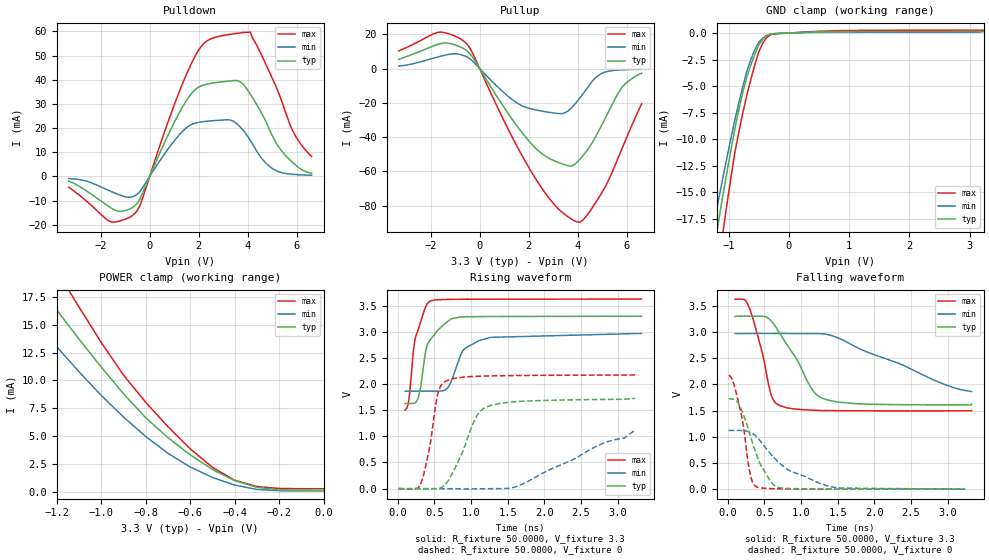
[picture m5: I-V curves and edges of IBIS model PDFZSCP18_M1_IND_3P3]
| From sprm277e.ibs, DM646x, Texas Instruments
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|   Model Cell PDFZSCP18_M1_IND_3P3
[Model]   PDFZSCP18_M1_IND_3P3
Model_type   I/O
Polarity   Non-Inverting
Enable   Active-Low
Vinl =  0.8V
Vinh =  2V
Cref =  10.0000pF
Rref =  50.0000
Vref =  1.5V
Vmeas =  1.65
C_comp   1.471252p   1.436302p   1.510805p
[Model Spec]
Vinl   0.8V   0.8V   0.8V
Vinh   2V   2V   2V
[Temperature Range]   25   125   -40
[Voltage Range]   3.3   2.97   3.63
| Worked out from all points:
|   slope of the pulldown table from 0 to 0.495 V, typ, clamps not added: 42.9 ohm
|   slope of the pullup table from 0 to 0.495 V, typ, clamps not added: 42.8 ohm
|   GND clamp passes 1 mA (typ) near -0.48 V on its own axis
|   POWER clamp passes 1 mA (typ) near -0.40 V on its own axis
|   rising waveform, R_fixture 50.0000, V_fixture 3.3: 20-80 % time 194ps typ, 261ps min, 145ps max; typ from 1.63 V to 3.3 V
|   rising waveform, R_fixture 50.0000, V_fixture 0: 20-80 % time 311ps typ, 973ps min, 153ps max; typ from 0 V to 1.73 V
|   falling waveform, R_fixture 50.0000, V_fixture 3.3: 20-80 % time 410ps typ, 1.11ns min, 214ps max; typ from 3.3 V to 1.63 V
|   falling waveform, R_fixture 50.0000, V_fixture 0: 20-80 % time 274ps typ, 623ps min, 153ps max; typ from 1.73 V to 0 V
[POWER_clamp]
|   voltage   I(typ)   I(min)   I(max)
-3.3V     84.79mA    64.06mA    102.5mA
-1.4V     21.98mA    17.8mA     26.67mA
-1.367V   21.02mA    17mA       25.54mA
-1.233V   17.27mA    13.84mA    21.04mA
-1.133V   14.62mA    11.55mA    17.73mA
-900mV    8.821mA    6.72mA     10.51mA
-800mV    6.658mA    4.97mA     8.044mA
-600mV    3.315mA    2.217mA    3.857mA
-500mV    1.994mA    1.273mA    2.187mA
-400mV    987.1uA    584.8uA    1.02mA
-300mV    389.1uA    194.4uA    453.4uA
0V        136.1uA    62.81uA    257uA
[Pulldown]
|   voltage   I(typ)   I(min)   I(max)
-3.3V     -1.945mA   -836.9uA   -4.474mA
-1.6V     -12.83mA   -6.075mA   -18.69mA
-600mV    -12.09mA   -8.013mA   -15.3mA
1.1V      24.29mA    15.95mA    32.25mA
1.9V      36.3mA     22.19mA    50.64mA
2.5V      38.52mA    23.01mA    56.95mA
3.3V      39.52mA    23.34mA    58.83mA
3.8V      38.23mA    19.26mA    59.54mA
4.1V      34.11mA    14.97mA    59.73mA
5V        16.81mA    3.301mA    40.55mA
5.9V      5.118mA    845.8uA    17.51mA
6.6V      1.393mA    503uA      8.266mA
[Pullup]
|   voltage   I(typ)   I(min)   I(max)
-3.3V     5.393mA    1.41mA     10.24mA
-1.7V     14.1mA     6.75mA     21.11mA
-600mV    11.14mA    7.267mA    15.41mA
-300mV    6.901mA    4.509mA    9.345mA
1.3V      -29.12mA   -17.81mA   -39.31mA
2.3V      -46.77mA   -24.19mA   -64.74mA
3.4V      -55.86mA   -26.23mA   -84.42mA
4V        -54.31mA   -18.73mA   -89.71mA
4.4V      -47.37mA   -11.08mA   -85.21mA
5.1V      -29.53mA   -2.142mA   -69.52mA
5.8V      -10.97mA   -782.4uA   -46.79mA
6.6V      -2.731mA   -431uA     -20.64mA
[GND_clamp]
|   voltage   I(typ)   I(min)   I(max)
-3.3V     -103.4mA   -79.15mA   -123mA
-1.3V     -22.54mA   -19.59mA   -27.1mA
-1.233V   -20.09mA   -17.63mA   -24.38mA
-1.167V   -17.72mA   -15.68mA   -21.67mA
-1.1V     -15.45mA   -13.76mA   -18.98mA
-1.033V   -13.3mA    -11.89mA   -16.36mA
-900mV    -9.149mA   -8.286mA   -11.38mA
-700mV    -4.193mA   -3.658mA   -5.925mA
-500mV    -1.139mA   -884.2uA   -1.786mA
-366.7mV  -266.6uA   -228.7uA   -433.6uA
700mV     116.3uA    56.08uA    197uA
3.233V    135.9uA    156.1uA    255uA
[Ramp]
| variable   typ   min   max
dV/dt_f  1.0171833/0.4162358n 0.71159794/1.1928752n   1.282012/0.21475807n
dV/dt_r  1.0420703/0.3127879n 0.69176769/1.0195835n  1.3118658/0.15395966n
R_load = 50
[Rising Waveform]
R_fixture = 50.0000
V_fixture = 3.3
V_fixture_min = 2.97
V_fixture_max = 3.63
|   time   V(typ)   V(min)   V(max)
99.98ps   1.627V     1.862V     1.5V
150.9ps   1.627V     1.863V     1.7V
242.3ps   1.647V     1.863V     2.893V
301.5ps   1.865V     1.863V     3.142V
393.4ps   2.699V     1.863V     3.516V
453.9ps   2.863V     1.863V     3.593V
745.6ps   3.252V     2.111V     3.619V
907.6ps   3.285V     2.669V     3.621V
1.259ns   3.292V     2.892V     3.623V
3.326ns   3.297V     2.968V     3.625V
[Rising Waveform]
R_fixture = 50.0000
V_fixture = 0
V_fixture_min = 0
V_fixture_max = 0
|   time   V(typ)   V(min)   V(max)
12.52ps   42.95uV    19.9uV     85.4uV
302.9ps   -2.844mV   25.53uV    65.61mV
414.8ps   -8.765mV   27.57uV    650.4mV
546.8ps   904.5uV    -63.04uV   1.814V
673.9ps   125mV      -1.432mV   2.066V
869.2ps   656.2mV    -5.709mV   2.129V
1.052ns   1.321V     -3.793mV   2.146V
1.195ns   1.552V     -1.728mV   2.153V
1.662ns   1.668V     64.14mV    2.163V
3.238ns   1.725V     1.121V     2.174V
[Falling Waveform]
R_fixture = 50.0000
V_fixture = 3.3
V_fixture_min = 2.97
V_fixture_max = 3.63
|   time   V(typ)   V(min)   V(max)
99.98ps   3.297V     2.968V     3.625V
219.8ps   3.301V     2.969V     3.623V
279.1ps   3.301V     2.97V      3.51V
456ps     3.299V     2.971V     2.683V
591.5ps   3.213V     2.97V      1.807V
700.4ps   2.997V     2.971V     1.601V
1.155ns   1.894V     2.97V      1.507V
1.304ns   1.728V     2.964V     1.501V
1.851ns   1.625V     2.647V     1.496V
3.326ns   1.627V     1.862V     1.5V
[Falling Waveform]
R_fixture = 50.0000
V_fixture = 0
V_fixture_min = 0
V_fixture_max = 0
|   time   V(typ)   V(min)   V(max)
12.52ps   1.725V     1.121V     2.174V
68.66ps   1.719V     1.121V     2.066V
159.5ps   1.599V     1.121V     1.586V
215ps     1.417V     1.116V     1.19V
303.4ps   1.04V      1.087V     309.1mV
391.9ps   662.9mV    1.003V     44.26mV
559.1ps   205.1mV    713.7mV    12.18mV
660.8ps   49.19mV    558.7mV    8.054mV
1.386ns   3.875mV    53.04mV    1.803mV
3.238ns   42.95uV    19.9uV     85.4uV
